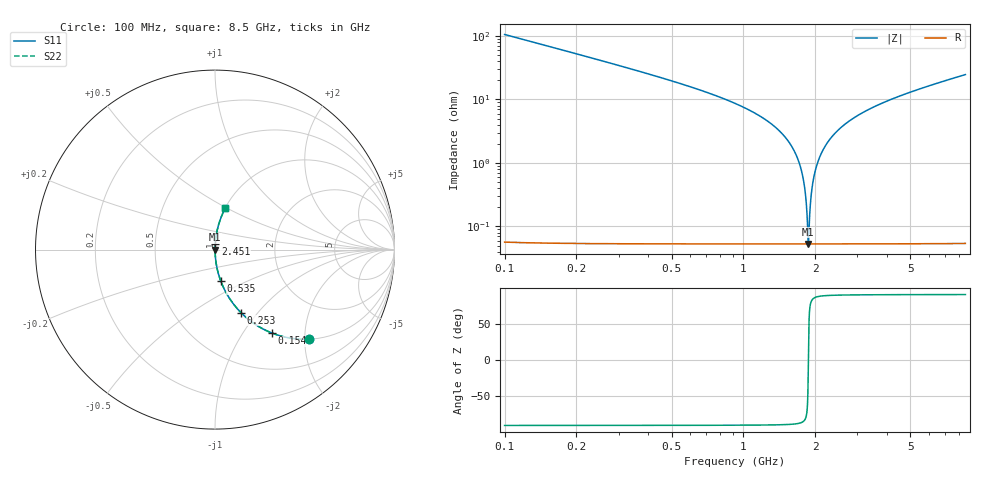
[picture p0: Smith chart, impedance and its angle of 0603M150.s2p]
! Created Wed Apr 18 16:40:06 2012
# hz S ma R 50
! 2 Port Network Data from SP1.SP block
! freq  magS11  angS11  magS21  angS21  magS12  angS12  magS22  angS22
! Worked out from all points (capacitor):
!   8401 points, 100 MHz to 8.5 GHz, reference 50 ohm
!   read as one part in series: C = 15 pF near 142 MHz
!   lowest |Z| = 53.2 mohm at 1.87 GHz (marker M1)
!   series resonance near 1.87 GHz, so ESL is about 480 pH
!   S11 on the Smith chart (normalised r, x): 100 MHz: 1.00, -2.11; 154 MHz: 1.00, -1.36; 253 MHz: 1.00, -0.82; 535 MHz: 1.00, -0.36; 2.451 GHz: 1.00, +0.06; 8.5 GHz: 1.00, +0.49
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1e8  0.7254 -43.5  0.6879 46.5  0.6879 46.5  0.7254 -43.5
1.54e8  0.5633 -55.7  0.8258 34.3  0.8258 34.3  0.5633 -55.7
2.53e8  0.3795 -67.6  0.9247 22.3  0.9247 22.3  0.3795 -67.6
5.35e8  0.1785 -79.6  0.9834 10.3  0.9834 10.3  0.1785 -79.6
1.222e9  0.04952 -86.5  0.9982 2.8  0.9982 2.8  0.04952 -86.5
1.5e9  0.02515 -87.3  0.9992 1.4  0.9992 1.4  0.02515 -87.3
1.639e9  0.01498 -87.1  0.9994 0.9  0.9994 0.9  0.01498 -87.1
1.737e9  0.008389 -85.9  0.9994 0.5  0.9994 0.5  0.008389 -85.9
1.791e9  0.004934 -83.5  0.9995 0.3  0.9995 0.3  0.004934 -83.5
1.843e9  0.00175 -72.2  0.9995 0.1  0.9995 0.1  0.00175 -72.2
1.87e9  0.0005319 -2.5  0.9995 0.0  0.9995 0.0  0.0005319 -2.5
1.897e9  0.001683 71.5  0.9995 -0.1  0.9995 -0.1  0.001683 71.5
1.931e9  0.003645 81.4  0.9995 -0.2  0.9995 -0.2  0.003645 81.4
1.96e9  0.00532 84.0  0.9995 -0.3  0.9995 -0.3  0.00532 84.0
2.048e9  0.01028 86.4  0.9994 -0.6  0.9994 -0.6  0.01028 86.4
2.209e9  0.01891 87.3  0.9993 -1.1  0.9993 -1.1  0.01891 87.3
2.451e9  0.03094 87.2  0.999 -1.8  0.999 -1.8  0.03094 87.2
2.9e9  0.05115 86.5  0.9982 -2.9  0.9982 -2.9  0.05115 86.5
4.3e9  0.105 83.7  0.9939 -6.0  0.9939 -6.0  0.105 83.7
5.7e9  0.1524 81.0  0.9878 -8.8  0.9878 -8.8  0.1524 81.0
7.1e9  0.1968 78.5  0.9799 -11.3  0.9799 -11.3  0.1968 78.5
8.5e9  0.2392 76.0  0.9704 -13.8  0.9704 -13.8  0.2392 76.0
